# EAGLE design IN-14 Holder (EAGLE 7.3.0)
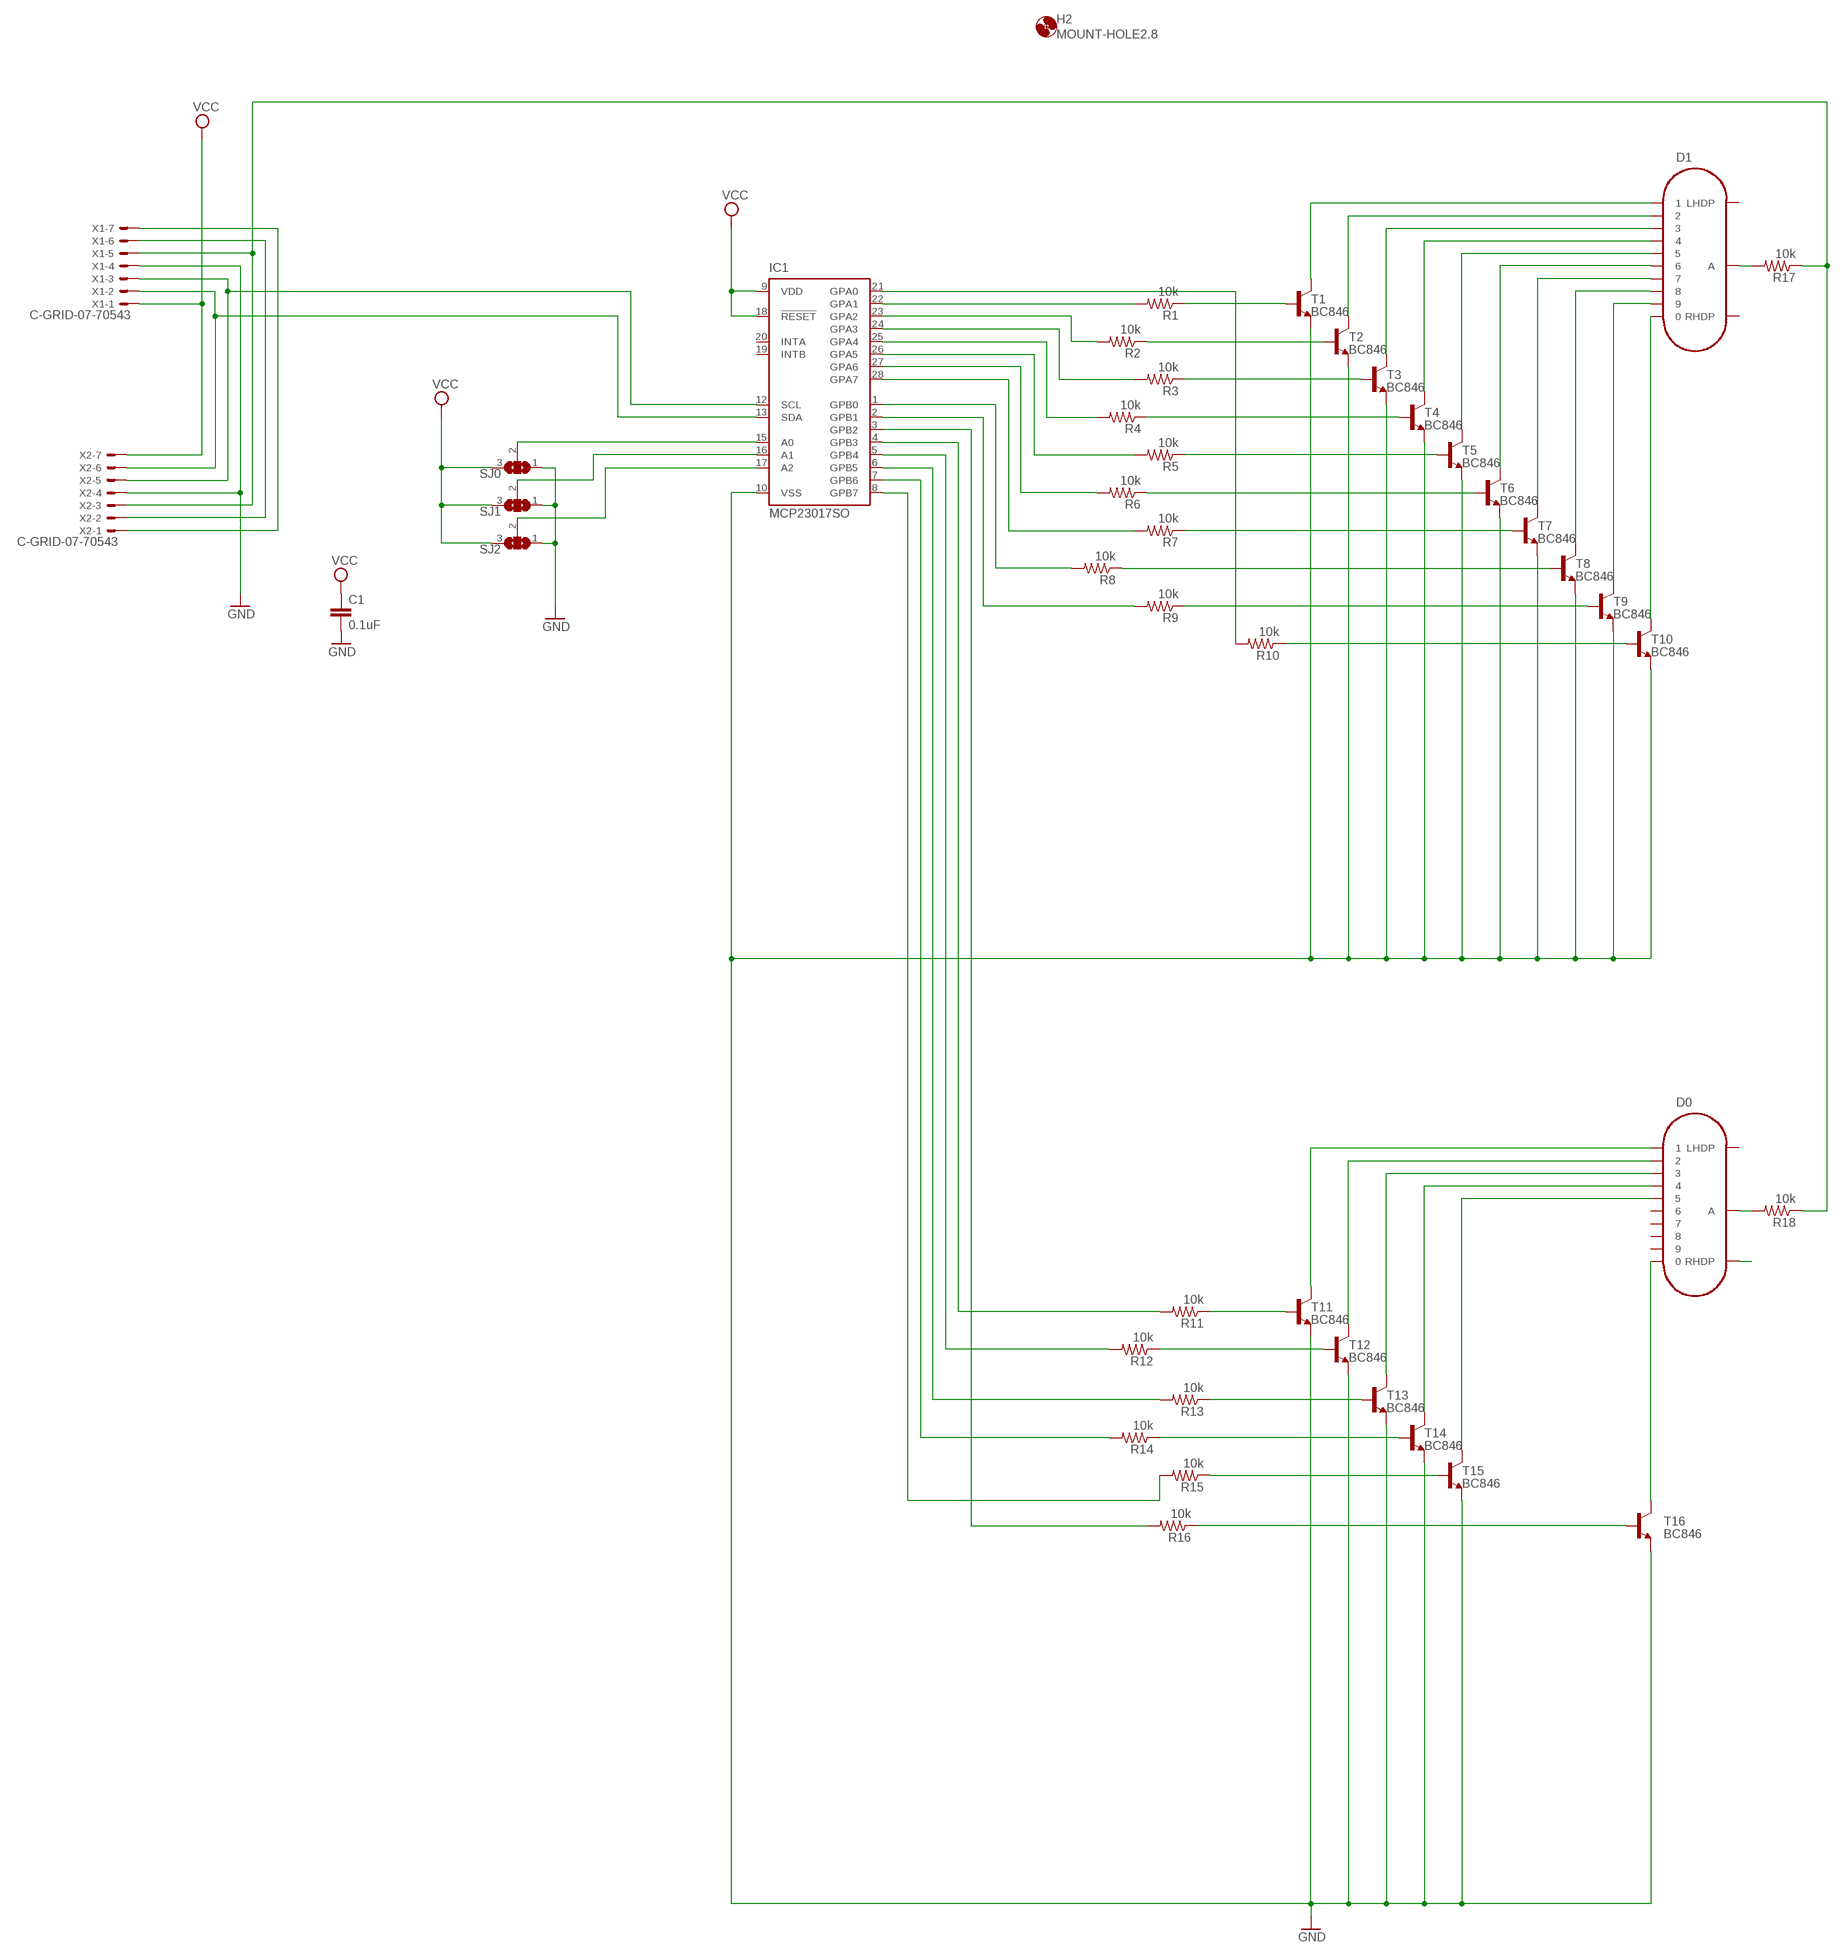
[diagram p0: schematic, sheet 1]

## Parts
C1  0.1uF  C-EUC1206  [C1206]
D0  IN-14  [IN-14]
D1  IN-14  [IN-14]
H2  MOUNT-HOLE2.8  [2,8]
IC1  MCP23017SO  [SO28W]
R1  10k  R-US_M0805  [M0805]
R2  10k  R-US_M0805  [M0805]
R3  10k  R-US_M0805  [M0805]
R4  10k  R-US_M0805  [M0805]
R5  10k  R-US_M0805  [M0805]
R6  10k  R-US_M0805  [M0805]
R7  10k  R-US_M0805  [M0805]
R8  10k  R-US_M0805  [M0805]
R9  10k  R-US_M0805  [M0805]
R10  10k  R-US_M0805  [M0805]
R11  10k  R-US_M0805  [M0805]
R12  10k  R-US_M0805  [M0805]
R13  10k  R-US_M0805  [M0805]
R14  10k  R-US_M0805  [M0805]
R15  10k  R-US_M0805  [M0805]
R16  10k  R-US_M0805  [M0805]
R17  10k  R-US_M0805  [M0805]
R18  10k  R-US_M0805  [M0805]
SJ0  SJ2W  [SJ_2]
SJ1  SJ2W  [SJ_2]
SJ2  SJ2W  [SJ_2]
T1  BC846  [SOT23]
T2  BC846  [SOT23]
T3  BC846  [SOT23]
T4  BC846  [SOT23]
T5  BC846  [SOT23]
T6  BC846  [SOT23]
T7  BC846  [SOT23]
T8  BC846  [SOT23]
T9  BC846  [SOT23]
T10  BC846  [SOT23]
T11  BC846  [SOT23]
T12  BC846  [SOT23]
T13  BC846  [SOT23]
T14  BC846  [SOT23]
T15  BC846  [SOT23]
T16  BC846  [SOT23]
X1  C-GRID-07-70543  [70543-07]
X2  C-GRID-07-70543  [70543-07]

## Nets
GND: C1.2 IC1.10(VSS) SJ0.1 SJ1.1 SJ2.1 T1.2(E) T2.2(E) T3.2(E) T4.2(E) T5.2(E) T6.2(E) T7.2(E) T8.2(E) T9.2(E) T10.2(E) T11.2(E) T12.2(E) T13.2(E) T14.2(E) T15.2(E) T16.2(E) X1.4 X2.4
N$1: IC1.15(A0) SJ0.2
N$2: R2.1 T2.1(B)
N$3: D1.1 T1.3(C)
N$4: R1.1 T1.1(B)
N$5: D1.2 T2.3(C)
N$6: D1.3 T3.3(C)
N$7: D1.4 T4.3(C)
N$8: D1.5 T5.3(C)
N$9: D0.A R18.2
N$10: R6.1 T6.1(B)
N$11: R7.1 T7.1(B)
N$12: IC1.22(GPA1) R1.2
N$13: D1.6 T6.3(C)
N$14: D1.A R17.2
N$15: D1.7 T7.3(C)
N$16: D1.8 T8.3(C)
N$17: D1.0 T10.3(C)
N$18: D1.9 T9.3(C)
N$19: IC1.24(GPA3) R3.2
N$20: IC1.25(GPA4) R4.2
N$21: IC1.26(GPA5) R5.2
N$22: IC1.27(GPA6) R6.2
N$23: R9.1 T9.1(B)
N$24: R8.1 T8.1(B)
N$25: R10.1 T10.1(B)
N$26: IC1.21(GPA0) R10.2
N$27: R16.1 T16.1(B)
N$28: R3.1 T3.1(B)
N$29: R15.1 T15.1(B)
N$30: R5.1 T5.1(B)
N$32: IC1.28(GPA7) R7.2
N$33: R14.1 T14.1(B)
N$34: IC1.5(GPB4) R12.2
N$37: IC1.2(GPB1) R9.2
N$38: R13.1 T13.1(B)
N$39: IC1.4(GPB3) R11.2
N$40: IC1.16(A1) SJ1.2
N$41: IC1.7(GPB6) R14.2
N$42: D0.3 T13.3(C)
N$43: IC1.17(A2) SJ2.2
N$45: D0.4 T14.3(C)
N$46: R12.1 T12.1(B)
N$47: R11.1 T11.1(B)
N$48: D0.5 T15.3(C)
N$50: X1.6 X2.2
N$51: X1.7 X2.1
N$52: IC1.8(GPB7) R15.2
N$53: IC1.3(GPB2) R16.2
N$54: IC1.6(GPB5) R13.2
N$55: D0.1 T11.3(C)
N$56: D0.2 T12.3(C)
N$58: D0.0 T16.3(C)
N$62: D0.RHDP
N$88: IC1.13(SDA) X1.2 X2.6
N$89: IC1.12(SCL) X1.3 X2.5
N$90: R17.1 R18.1 X1.5 X2.3
R: R4.1 T4.1(B)
R2: IC1.23(GPA2) R2.2
R14: IC1.1(GPB0) R8.2
VCC: C1.1 IC1.9(VDD) IC1.18(!RESET) SJ0.3 SJ1.3 SJ2.3 X1.1 X2.7
Unconnected: D0.6 D0.7 D0.8 D0.9 D0.LHDP D1.LHDP D1.RHDP IC1.19(INTB) IC1.20(INTA)

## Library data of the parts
C1 = rcl:C-EU: CAPACITOR, European symbol
D0 D1 = russian-nixies:IN-14: IN-14: medium numeric frontview nixie tube
H2 = holes:MOUNT-HOLE: MOUNTING HOLE with drill center marker
IC1 = adafruit:MCP23017: http://ww1.microchip.com/downloads/en/DeviceDoc/21952a.pdf Source: http://ww1.microchip.com/downloads/en/DeviceDoc/21952a.pdf
R1-R18 = adafruit:R-US_: RESISTOR, American symbol
SJ0 SJ1 SJ2 = jumper:SJ2W: SMD solder JUMPER
T1-T16 = transistor:BC846: NPN TRANSISTOR
X1 X2 = con-molex:C-GRID-07: CONNECTOR wire to board 2.54 mm (0.100") pitch header; OC_FARNELL: unknown; OC_NEWARK: unknown

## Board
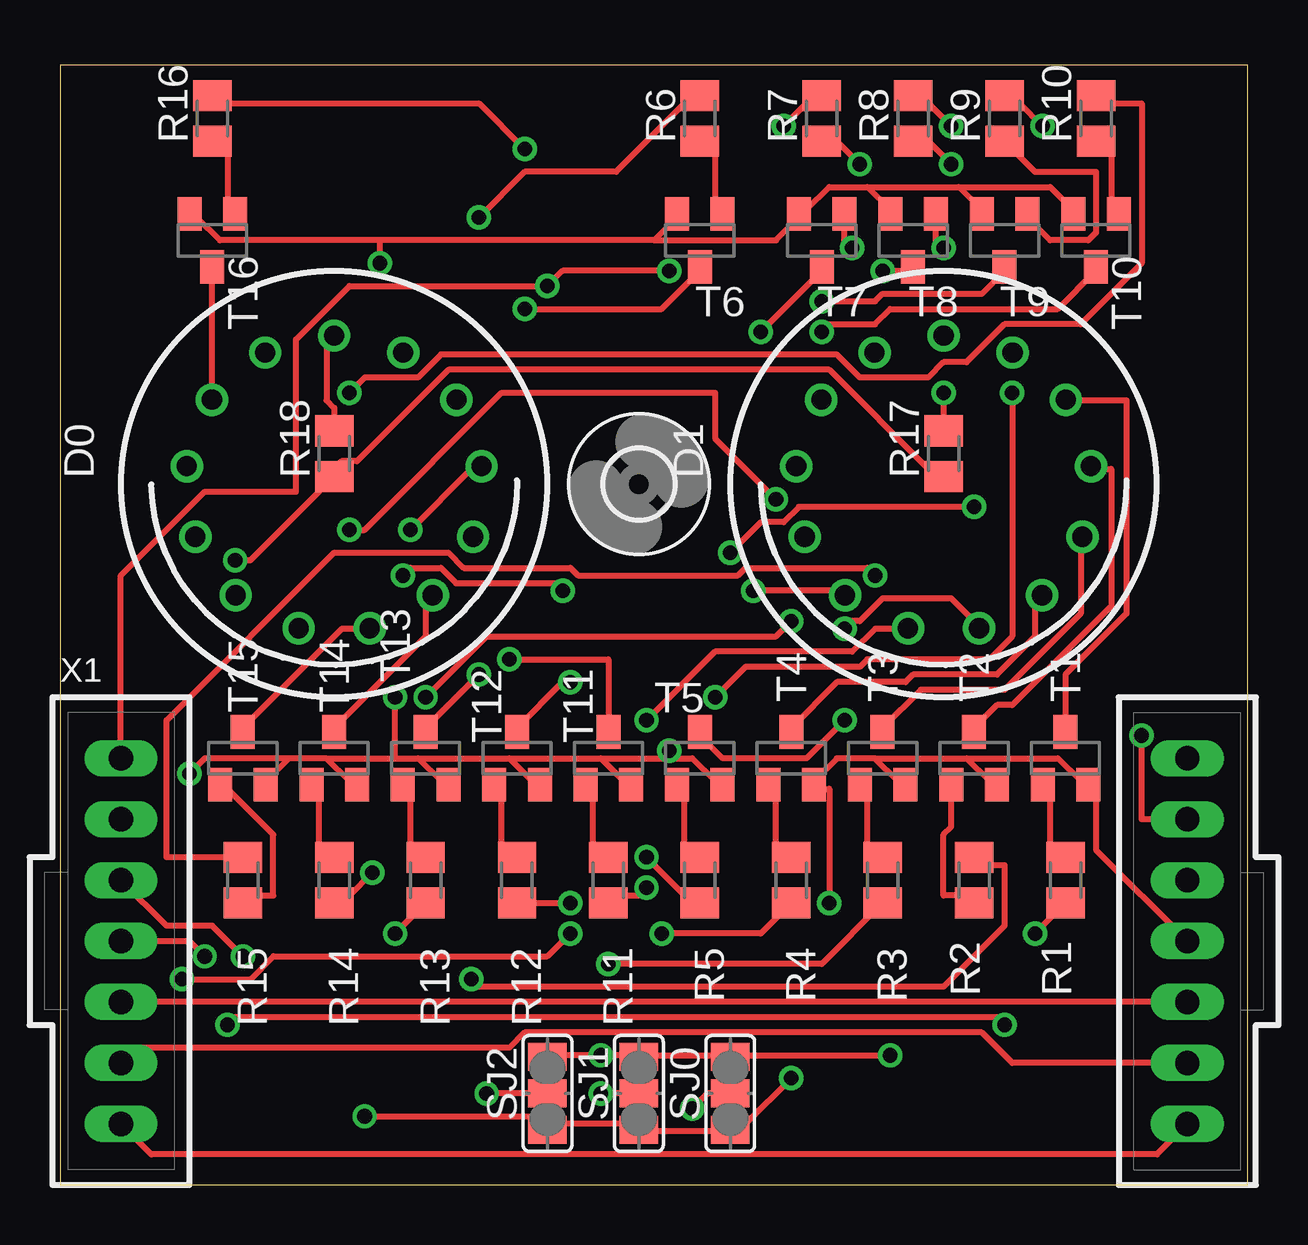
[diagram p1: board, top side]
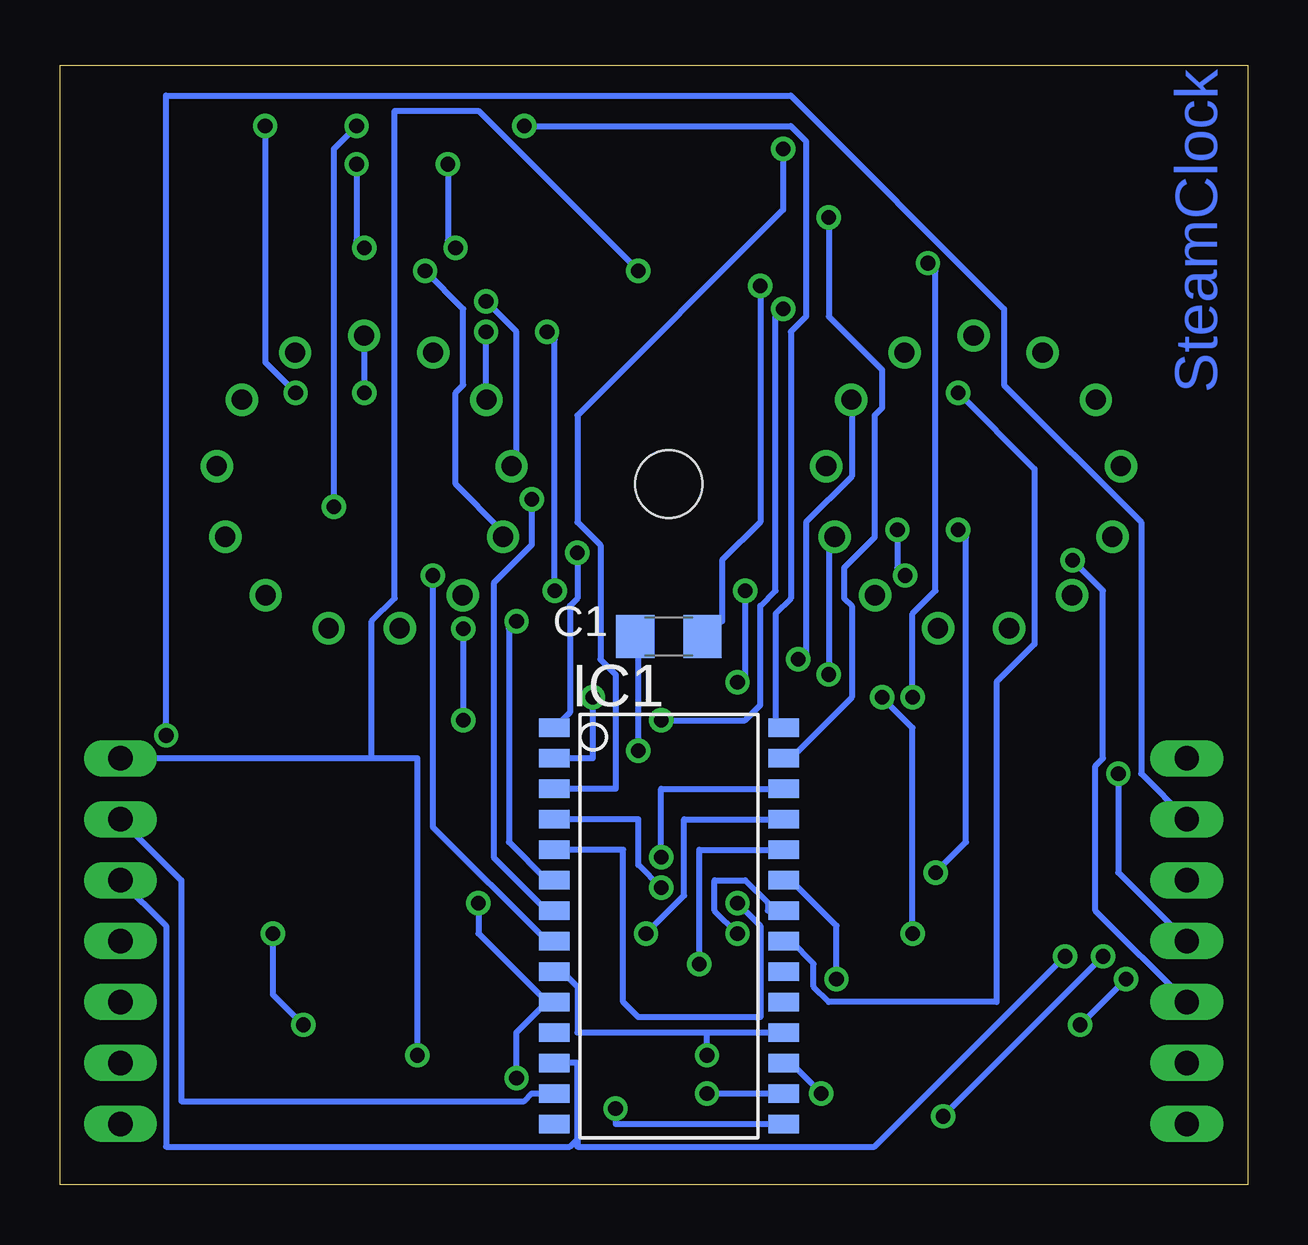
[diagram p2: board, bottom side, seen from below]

Size 49.51 x 46.66 mm. Coordinates in mm from the lower left corner, seen from the top.
Outline: 0,0 49.51,0 49.51,46.66 0,46.66 0,0
Copper layers (1*16): Top 0.035mm / dielectric 1.5mm / Bottom 0.035mm
Design rules "default": minimum track width 10mil, minimum drill 24mil, track to track 8mil, track to pad 8mil, pad to pad 8mil, via to via 8mil, smd to smd 8mil, copper to edge 40mil, drill to drill 8mil, minimum pad ring 10mil, minimum via ring 8mil, stop-mask expansion 4mil, vias tented up to drill 0mil, thermal gap 10mil

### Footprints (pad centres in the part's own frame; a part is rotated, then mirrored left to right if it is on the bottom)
C1206 = smd 1.6 x 1.8: 1 -1.4,0; 2 1.4,0
IN-14 = drill 0.84: 0 5.094,-3.516; 1 -5.094,-3.516; 2 -6.145,-0.746; 3 -5.788,2.195; 4 -4.105,4.633; 5 -1.481,6.01; 6 1.481,6.01; 7 4.105,4.633; 8 5.788,2.195; 9 6.145,-0.746; A 0,-6.19; LHDP 2.877,-5.481; RHDP -2.877,-5.481
2,8 = hole 2.8: 0,0
SO28W = smd 0.762 x 1.27: 1 -7.62,-4.78; 2 -6.35,-4.78; 3 -5.08,-4.78; 4 -3.81,-4.78; 5 -2.54,-4.78; 6 -1.27,-4.78; 7 0,-4.78; 8 1.27,-4.78; 9 2.54,-4.78; 10 3.81,-4.78; 11 5.08,-4.78; 12 6.35,-4.78; 13 7.62,-4.78; 14 8.89,-4.78; 15 8.89,4.78; 16 7.62,4.78; 17 6.35,4.78; 18 5.08,4.78; 19 3.81,4.78; 20 2.54,4.78; 21 1.27,4.78; 22 0,4.78; 23 -1.27,4.78; 24 -2.54,4.78; 25 -3.81,4.78; 26 -5.08,4.78; 27 -6.35,4.78; 28 -7.62,4.78
M0805 = smd 1.3 x 1.6: 1 -0.95,0; 2 0.95,0
SJ_2 = smd 1.168 x 1.6: 1 -1.524,0; 2 0,0; 3 1.524,0
SOT23 = smd 1 x 1.4: 1 -0.95,-1.1; 2 0.95,-1.1; 3 0,1.1
70543-07 = drill 1.016 long: 1 -7.62,0; 2 -5.08,0; 3 -2.54,0; 4 0,0; 5 2.54,0; 6 5.08,0; 7 7.62,0

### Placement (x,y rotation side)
C1  24.13,22.86 180 bottom
D0  11.43,29.21 180 top
D1  36.83,29.21 180 top
H2  24.13,29.21 0 top
IC1  24.13,11.43 270 bottom
R1  41.91,12.7 270 top
R2  38.1,12.7 90 top
R3  34.29,12.7 270 top
R4  30.48,12.7 270 top
R5  26.67,12.7 270 top
R6  26.67,44.45 90 top
R7  31.75,44.45 90 top
R8  35.56,44.45 90 top
R9  39.37,44.45 90 top
R10  43.18,44.45 90 top
R11  22.86,12.7 270 top
R12  19.05,12.7 270 top
R13  15.24,12.7 270 top
R14  11.43,12.7 270 top
R15  7.62,12.7 90 top
R16  6.35,44.45 90 top
R17  36.83,30.48 90 top
R18  11.43,30.48 90 top
SJ0  27.94,3.81 90 top
SJ1  24.13,3.81 90 top
SJ2  20.32,3.81 90 top
T1  41.91,17.78 0 top
T2  38.1,17.78 0 top
T3  34.29,17.78 0 top
T4  30.48,17.78 0 top
T5  26.67,17.78 0 top
T6  26.67,39.37 180 top
T7  31.75,39.37 180 top
T8  35.56,39.37 180 top
T9  39.37,39.37 180 top
T10  43.18,39.37 180 top
T11  22.86,17.78 0 top
T12  19.05,17.78 0 top
T13  15.24,17.78 0 top
T14  11.43,17.78 0 top
T15  7.62,17.78 0 top
T16  6.35,39.37 180 top
X1  2.54,10.16 270 top
X2  46.99,10.16 90 top

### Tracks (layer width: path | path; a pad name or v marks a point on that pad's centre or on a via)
GND  (via drill 0.61)
  Top 0.254: 20.32,2.54 24.13,2.54 SJ1.1 24.13,2.22 27.94,2.22 SJ0.1 27.94,2.54 28.57,2.54 v30.48,4.45 | 33.97,17.78 32.38,17.78 31.43,16.83 T4.2 31.43,16.51 32.07,16.51 v32.07,11.75 | 33.97,17.78 34.92,16.83 T3.2 | 37.78,17.78 38.73,16.83 T2.2 | 33.97,17.78 37.78,17.78 | 37.78,17.78 41.59,17.78 42.55,16.83 T1.2 42.86,16.51 43.18,16.51 43.18,13.97 X2.4 | 24.77,39.37 13.34,39.37 | 13.34,39.37 6.67,39.37 5.71,40.32 T16.2 | 24.77,39.37 25.72,40.32 T6.2 | 24.77,39.37 29.84,39.37 30.8,40.32 T7.2 31.11,40.64 32.07,41.59 33.66,41.59 | 33.66,41.59 34.61,40.64 T8.2 | 37.47,41.59 38.42,40.64 T9.2 | 33.66,41.59 37.47,41.59 | 37.47,41.59 41.27,41.59 42.23,40.64 T10.2 | 9.53,17.78 8.57,16.83 T15.2 | 11.11,17.78 9.53,17.78 | 11.11,17.78 12.06,16.83 T14.2 | 14.92,17.78 15.88,16.83 T13.2 | 11.11,17.78 13.97,17.78 | 13.97,17.78 14.92,17.78 | 18.73,17.78 19.68,16.83 T12.2 | 14.92,17.78 18.73,17.78 | 22.54,17.78 23.5,16.83 T11.2 | 18.73,17.78 22.54,17.78 | 22.54,17.78 25.4,17.78 | 25.4,17.78 26.35,17.78 27.3,16.83 T5.2 | 25.4,17.78 v25.4,18.1 | v5.4,17.14 6.03,17.78 9.53,17.78 | v13.34,38.42 13.34,39.37 | 13.97,17.78 v13.97,20.32 | 20.32,2.54 20,2.86 v12.7,2.86 | v6.03,9.53 5.4,10.16 X1.4 | 20.32,2.54 SJ2.1
  Bottom 0.254: 29.21,7.62 30.48,6.35 v30.48,4.45 | 29.21,7.62 32.07,10.48 v32.07,11.75 | 29.21,7.62 IC1.10 | v25.4,18.1 25.4,22.86 C1.2 | X1.4 5.4,13.02 v5.4,17.14 | v13.34,38.42 13.02,38.1 13.02,24.77 13.97,23.81 v13.97,20.32 | v6.03,9.53 v12.7,2.86
N$1  (via drill 0.61)
  Top 0.254: v26.35,3.17 26.99,3.81 SJ0.2
  Bottom 0.254: IC1.15 26.35,2.54 v26.35,3.17
N$2
  Top 0.254: T2.1 37.15,16.51 37.15,14.92 36.83,14.61 36.83,12.06 38.1,12.06 R2.1
N$3
  Top 0.254: T1.3 41.91,21.27 44.45,23.81 44.45,32.7 42.23,32.7 D1.1
N$4
  Top 0.254: T1.1 41.27,16.51 41.27,13.65 R1.1
N$5
  Top 0.254: T2.3 38.1,19.05 39.05,20 39.69,20 43.81,24.13 43.81,29.84 43.18,29.84 D1.2
N$6
  Top 0.254: T3.3 34.29,19.05 35.88,20.64 39.37,20.64 42.55,23.81 42.55,26.99 D1.3
N$7
  Top 0.254: T4.3 30.48,19.05 32.38,20.95 35.24,20.95 35.56,21.27 39.05,21.27 40.64,22.86 40.64,24.45 D1.4
N$8  (via drill 0.61)
  Top 0.254: v32.7,19.37 31.11,17.78 27.62,17.78 26.67,18.73 T5.3 | v32.7,23.18 33.02,23.5 33.34,23.5 34.29,24.45 37.15,24.45 38.1,23.5 D1.5
  Bottom 0.254: v32.7,23.18 v32.7,19.37
N$9
  Top 0.254: R18.2 11.43,32.38 11.11,32.7 11.11,35.24 11.43,35.24 D0.A
N$10
  Top 0.254: T6.1 27.3,40.64 27.3,43.5 R6.1
N$11  (via drill 0.61)
  Top 0.254: v33.02,39.05 32.7,39.05 32.7,40.32 T7.1 | v33.34,42.55 32.38,43.5 R7.1
  Bottom 0.254: v33.02,39.05 33.34,39.37 v33.34,42.55
N$12  (via drill 0.61)
  Top 0.254: v21.27,10.48 20.32,9.53 8.89,9.53 7.94,8.57 v5.08,8.57 | v6.99,6.67 7.3,6.99 39.05,6.99 v39.37,6.67 | v40.64,10.48 R1.2
  Bottom 0.254: IC1.22 20,11.43 20,11.75 20.95,12.7 22.23,12.7 22.23,11.43 v21.27,10.48 | v6.99,6.67 v5.08,8.57 | v39.37,6.67 40.64,7.94 v40.64,10.48
N$13  (via drill 0.61)
  Top 0.254: v19.37,36.51 25.08,36.51 26.67,38.1 T6.3 | v24.45,19.37 27.3,22.23 33.02,22.23 33.97,23.18 35.24,23.18 D1.6
  Bottom 0.254: v19.37,36.51 19.68,36.2 19.68,24.77 20.32,24.13 20.32,20 20.95,19.37 v24.45,19.37
N$14  (via drill 0.61)
  Top 0.254: v36.83,33.02 R17.2
  Bottom 0.254: D1.A v36.83,33.02
N$15  (via drill 0.61)
  Top 0.254: v29.21,35.56 31.75,38.1 T7.3 | v28.89,24.77 32.7,24.77 D1.7
  Bottom 0.254: v29.21,35.56 28.89,35.24 v28.89,24.77
N$16  (via drill 0.61)
  Top 0.254: v34.29,38.1 35.56,38.1 T8.3
  Bottom 0.254: v34.29,38.1 32.7,36.51 32.7,33.34 33.02,33.02 33.02,29.21 31.11,27.3 D1.8
N$17  (via drill 0.61)
  Top 0.254: v31.75,35.56 32.07,35.88 33.97,35.88 34.61,36.51 41.59,36.51 43.18,38.1 T10.3
  Bottom 0.254: v31.75,35.56 31.75,33.02 D1.0
N$18  (via drill 0.61)
  Top 0.254: v31.75,36.83 33.97,36.83 34.29,37.15 38.42,37.15 39.37,38.1 T9.3
  Bottom 0.254: v31.75,36.83 30.48,35.56 30.48,30.16 D1.9
N$19  (via drill 0.61)
  Top 0.254: v22.86,9.21 31.75,9.21 R3.2
  Bottom 0.254: IC1.24 22.86,13.97 v22.86,9.21
N$20  (via drill 0.61)
  Top 0.254: v25.08,10.48 29.21,10.48 R4.2
  Bottom 0.254: IC1.25 23.5,15.24 23.5,12.06 v25.08,10.48
N$21  (via drill 0.61)
  Top 0.254: v24.45,13.65 26.04,12.06 26.67,12.06 R5.2
  Bottom 0.254: IC1.26 24.45,16.51 v24.45,13.65
N$22  (via drill 0.61)
  Top 0.254: v17.46,40.32 19.37,42.23 23.18,42.23 26.04,45.09 26.67,45.09 R6.2
  Bottom 0.254: v17.46,40.32 17.46,36.2 15.24,33.97 15.24,32.38 15.56,32.07 15.56,26.99 16.83,25.72 16.83,24.45 16.51,24.13 16.51,20.32 19.05,17.78 IC1.27
N$23
  Top 0.254: T9.1 40.32,40.32 41.27,39.37 42.86,39.37 43.18,39.69 43.18,42.23 40.64,42.23 R9.1
N$24  (via drill 0.61)
  Top 0.254: v36.83,39.05 36.51,39.05 36.51,40.32 T8.1 | v37.15,42.55 36.2,43.5 R8.1
  Bottom 0.254: v36.83,39.05 37.15,39.37 v37.15,42.55
N$25
  Top 0.254: T10.1 43.81,40.64 43.81,43.5 R10.1
N$26  (via drill 0.61)
  Top 0.254: v12.06,33.02 12.7,33.66 14.92,33.66 15.88,34.61 32.38,34.61 33.34,33.66 36.2,33.66 36.83,34.29 37.78,34.29 39.37,35.88 42.55,35.88 45.09,38.42 45.09,45.09 43.18,45.09 R10.2
  Bottom 0.254: v12.06,33.02 8.89,29.84 8.89,22.54 10.48,20.95 10.48,7.62 17.46,7.62 18.1,8.26 18.1,9.21 19.05,10.16 IC1.21
N$27
  Top 0.254: T16.1 6.99,40.64 6.99,43.5 R16.1
N$28
  Top 0.254: T3.1 33.66,16.51 33.66,13.65 R3.1
N$29
  Top 0.254: T15.1 6.99,16.51 8.89,14.61 8.89,12.06 7.62,12.06 R15.1
N$30
  Top 0.254: T5.1 26.04,16.51 26.04,13.65 R5.1
N$32  (via drill 0.61)
  Top 0.254: v30.16,44.13 31.11,45.09 31.75,45.09 R7.2
  Bottom 0.254: v30.16,44.13 19.05,44.13 18.41,43.5 18.41,36.2 19.05,35.56 19.05,24.45 19.68,23.81 19.68,19.37 19.37,19.05 IC1.28
N$33
  Top 0.254: T14.1 10.79,16.51 10.79,13.65 R14.1
N$34  (via drill 0.61)
  Top 0.254: v21.27,11.75 R12.2
  Bottom 0.254: IC1.5 26.04,13.97 26.04,7.62 25.4,6.99 20.32,6.99 20.32,10.79 v21.27,11.75
N$37  (via drill 0.61)
  Top 0.254: v27.3,20.32 28.57,21.59 33.34,21.59 33.66,21.91 38.73,21.91 39.69,22.86 v39.69,33.02 | v40.96,44.13 40.01,45.09 39.37,45.09 R9.2
  Bottom 0.254: IC1.2 27.3,17.78 v27.3,20.32 | v39.69,33.02 40.96,34.29 v40.96,44.13
N$38
  Top 0.254: T13.1 14.61,16.51 14.61,13.65 R13.1
N$39  (via drill 0.61)
  Top 0.254: v24.45,12.38 24.13,12.06 22.86,12.06 R11.2
  Bottom 0.254: IC1.4 25.4,15.24 25.4,13.34 v24.45,12.38
N$40  (via drill 0.61)
  Top 0.254: SJ1.2 v22.54,3.81
  Bottom 0.254: v22.54,3.81 IC1.16
N$41  (via drill 0.61)
  Top 0.254: v29.84,28.57 27.3,31.11 27.3,33.02 18.41,33.02 12.7,27.3 v12.06,27.3 | v13.02,13.02 12.06,12.06 11.43,12.06 R14.2
  Bottom 0.254: v29.84,28.57 29.84,26.67 31.43,25.08 31.43,13.65 29.21,11.43 IC1.7 | v12.06,27.3 11.75,26.99 11.75,14.29 v13.02,13.02
N$42  (via drill 0.61)
  Top 0.254: v17.46,21.27 15.24,19.05 T13.3
  Bottom 0.254: v17.46,21.27 17.46,26.99 D0.3
N$43  (via drill 0.61)
  Top 0.254: SJ2.2 v17.78,3.81
  Bottom 0.254: v17.78,3.81 19.05,5.08 IC1.17
N$45
  Top 0.254: T14.3 11.43,19.05 15.24,22.86 15.24,24.45 D0.4
N$46
  Top 0.254: T12.1 18.41,16.51 18.41,13.65 R12.1
N$47
  Top 0.254: T11.1 22.23,16.51 22.23,13.65 R11.1
N$48
  Top 0.254: T15.3 7.62,19.05 11.75,23.18 12.7,23.18 D0.5
N$50
  Top 0.254: X1.6 3.17,5.71 18.73,5.71 19.37,6.35 38.42,6.35 39.69,5.08 X2.2
N$51
  Top 0.254: X1.7 3.81,1.27 45.72,1.27 X2.1
N$52  (via drill 0.61)
  Top 0.254: v33.97,25.4 33.66,25.72 28.57,25.72 28.26,25.4 21.59,25.4 21.27,25.72 16.83,25.72 16.19,26.35 11.43,26.35 4.45,19.37 4.45,13.65 R15.2
  Bottom 0.254: v33.97,25.4 33.97,14.92 29.21,10.16 IC1.8
N$53  (via drill 0.61)
  Top 0.254: v19.37,43.18 17.46,45.09 6.35,45.09 R16.2
  Bottom 0.254: IC1.3 26.35,16.51 26.35,21.27 26.99,21.91 26.99,26.67 27.94,27.62 27.94,32.07 19.37,40.64 v19.37,43.18
N$54  (via drill 0.61)
  Top 0.254: v30.48,23.5 29.84,22.86 17.78,22.86 v15.24,20.32 | v13.97,10.48 R13.2
  Bottom 0.254: v30.48,23.5 30.8,23.18 30.8,14.29 29.21,12.7 IC1.6 | v15.24,20.32 13.97,19.05 v13.97,10.48
N$55  (via drill 0.61)
  Top 0.254: T11.3 22.86,21.91 v18.73,21.91
  Bottom 0.254: v18.73,21.91 18.41,22.23 18.41,27.62 16.51,29.53 16.51,32.7 D0.1
N$56  (via drill 0.61)
  Top 0.254: v21.27,20.95 20.95,20.95 19.05,19.05 T12.3 | v20.95,24.77 20.64,25.08 16.51,25.08 15.88,25.72 14.61,25.72 v14.29,25.4 | v14.61,27.3 17.14,29.84 17.46,29.84 D0.2
  Bottom 0.254: v21.27,20.95 20.95,21.27 v20.95,24.77 | v14.29,25.4 14.61,25.72 v14.61,27.3
N$58
  Top 0.254: T16.3 6.35,33.02 D0.0
N$88  (via drill 0.61)
  Top 0.254: v45.09,18.73 45.09,15.24 X2.6
  Bottom 0.254: IC1.13 29.84,3.81 30.16,3.49 44.45,3.49 44.45,12.7 X2.6 | X1.2 4.45,17.14 4.45,27.62 10.16,33.34 10.16,36.51 19.05,45.4 45.09,45.4 v45.09,18.73
N$89  (via drill 0.61)
  Top 0.254: X1.3 4.45,10.79 6.35,10.79 v7.62,9.53
  Bottom 0.254: IC1.12 27.94,5.08 27.94,1.91 | 27.94,1.91 28.26,1.59 45.09,1.59 45.09,10.79 X2.5 | v7.62,9.53 15.56,1.59 27.94,1.59 27.94,1.91
N$90  (via drill 0.61)
  Top 0.254: R17.1 36.83,29.84 36.2,29.84 32.07,33.97 16.19,33.97 12.38,30.16 11.75,30.16 11.43,29.84 R18.1 7.94,26.04 v7.3,26.04 | X2.3 X1.5
  Bottom 0.254: v7.3,26.04 6.03,24.77 6.03,17.78 6.35,17.46 6.35,11.43 X1.5
R
  Top 0.254: T4.1 29.84,16.51 29.84,13.65 R4.1
R2  (via drill 0.61)
  Top 0.254: v17.14,8.57 17.46,8.26 36.83,8.26 39.37,10.79 39.37,13.34 38.1,13.34 R2.2
  Bottom 0.254: v17.14,8.57 17.14,10.79 19.05,12.7 IC1.23
R14  (via drill 0.61)
  Top 0.254: v27.94,26.35 29.21,27.62 30.16,27.62 30.8,28.26 v38.1,28.26 | v37.15,44.13 36.2,45.09 35.56,45.09 R8.2
  Bottom 0.254: v27.94,26.35 27.94,24.45 28.26,24.13 28.26,19.68 28.89,19.05 IC1.1 | v38.1,28.26 38.1,43.18 v37.15,44.13
VCC  (via drill 0.61)
  Top 0.254: X1.1 2.54,25.4 6.03,28.89 9.84,28.89 9.84,35.24 12.06,37.47 v20.32,37.47 20.95,38.1 v25.4,38.1 | 24.13,5.4 v22.54,5.4 20.32,5.4 SJ2.3 | 24.13,5.4 27.94,5.4 | 24.13,5.4 SJ1.3 | 27.94,5.4 v34.61,5.4 | 27.94,5.4 SJ0.3
  Bottom 0.254: v20.32,37.47 20.32,27.62 21.91,26.04 21.91,23.5 22.54,22.86 C1.1 | 22.54,6.35 27.94,6.35 27.94,8.26 28.57,8.89 IC1.9 | 22.54,6.35 IC1.18 | 36.51,17.78 34.61,17.78 v34.61,5.4 | 36.51,17.78 X2.7 | v22.54,5.4 22.54,6.35 | v25.4,38.1 32.07,44.77 35.56,44.77 35.56,24.45 36.51,23.5 36.51,17.78

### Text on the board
Bottom: SteamClock | SteamClock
